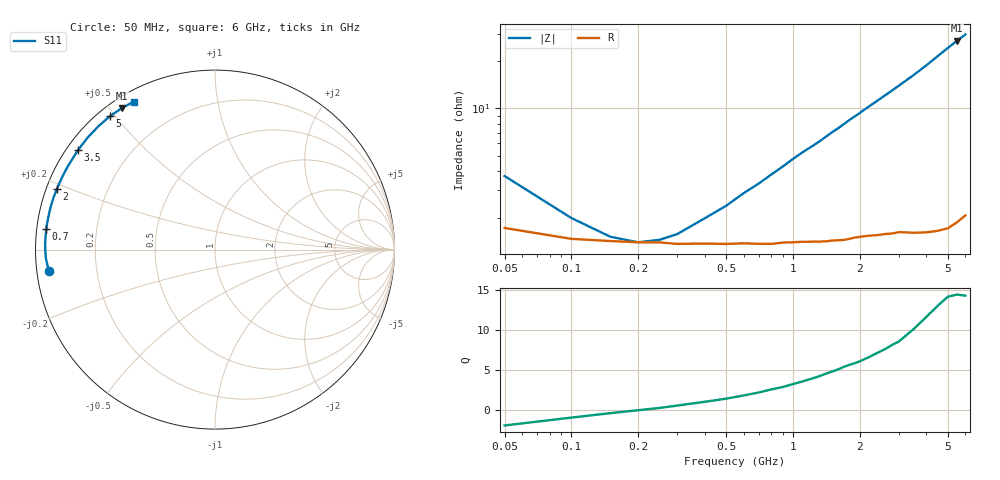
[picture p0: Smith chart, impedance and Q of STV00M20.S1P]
! SIEMENS Discrete & RF Semiconductors
! BA892
! Si PIN Diode in SCD-80
! IF = 0.2 mA
! S-Parameters:  September  1997
# GHz  S  MA  R  50
!  f  S11
! GHz  MAG  ANG
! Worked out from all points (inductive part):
!   34 points, 50 MHz to 6 GHz, reference 50 ohm
!   read as one part to ground: L = 727 pH near 1 GHz
!   highest Q = 14.3 at 5.5 GHz (marker M1), where L = 781 pH
!   S11 on the Smith chart (normalised r, x): 50 MHz: 0.03, -0.07; 700 MHz: 0.03, +0.06; 2 GHz: 0.03, +0.18; 3.5 GHz: 0.03, +0.32; 5 GHz: 0.03, +0.49; 6 GHz: 0.04, +0.59
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0.05  0.9336 -172.5
0.1  0.943 -176.9
0.15  0.9447 -178.8
0.2  0.9456 180.0
0.3  0.9469 178.2
0.4  0.9467 176.7
0.5  0.947 175.5
0.6  0.9466 174.2
0.7  0.947 173.1
0.8  0.9472 171.9
0.9  0.9462 170.8
1  0.9461 169.6
1.1  0.9458 168.5
1.3  0.9458 166.5
1.5  0.9453 164.3
1.6  0.9452 163.3
1.8  0.9444 161.1
2  0.9431 159.1
2.2  0.9426 157.0
2.4  0.9426 155.0
2.8  0.9422 151.0
3  0.9415 149.0
3.5  0.9435 144.0
4  0.9449 138.8
4.5  0.9457 133.4
5  0.946 128.2
5.5  0.9436 123.2
6  0.9404 118.7
